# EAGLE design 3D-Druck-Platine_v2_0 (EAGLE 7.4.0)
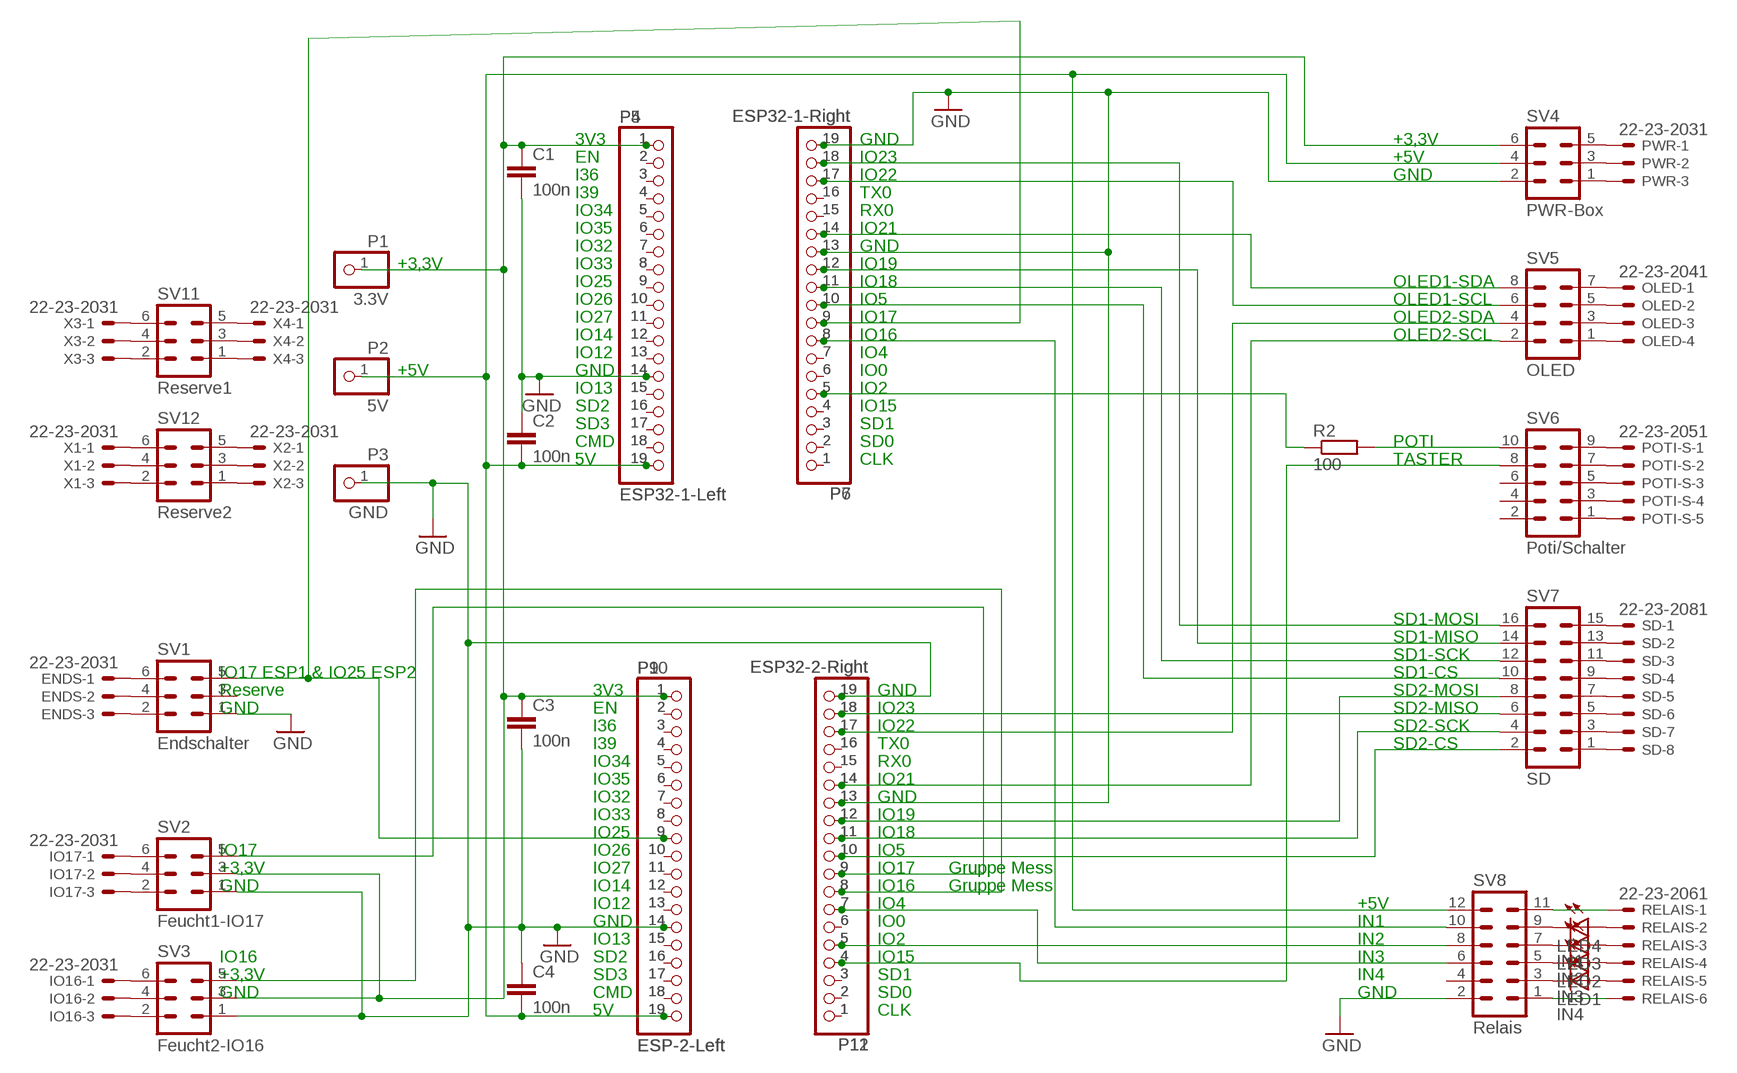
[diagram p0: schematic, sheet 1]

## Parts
C1  100n  C-EU025-024X044  [C025-024X044]
C2  100n  C-EU025-024X044  [C025-024X044]
C3  100n  C-EU025-024X044  [C025-024X044]
C4  100n  C-EU025-024X044  [C025-024X044]
ENDS  22-23-2031  [22-23-2031]
IO16  22-23-2031  [22-23-2031]
IO17  22-23-2031  [22-23-2031]
LED1  IN4  LED3MM  [LED3MM]
LED2  IN3  LED3MM  [LED3MM]
LED3  IN2  LED3MM  [LED3MM]
LED4  IN1  LED3MM  [LED3MM]
OLED  22-23-2041  [22-23-2041]
P1  3.3V  PINHD-1X1  [1X01]
P2  5V  PINHD-1X1  [1X01]
P3  GND  PINHD-1X1  [1X01]
P4  ESP32-1-Left  PINHD-1X19  [1X19]
P5  ESP32-1-Left  PINHD-1X19  [1X19]
P6  ESP32-1-Right  PINHD-1X19  [1X19]
P7  ESP32-1-Right  PINHD-1X19  [1X19]
P9  ESP-2-Left  PINHD-1X19  [1X19]
P10  ESP-2-Left  PINHD-1X19  [1X19]
P11  ESP32-2-Right  PINHD-1X19  [1X19]
P12  ESP32-2-Right  PINHD-1X19  [1X19]
POTI-S  22-23-2051  [22-23-2051]
PWR  22-23-2031  [22-23-2031]
R2  100  R-EU_0207/10  [0207/10]
RELAIS  22-23-2061  [22-23-2061]
SD  22-23-2081  [22-23-2081]
SV1  Endschalter  MA03-2  [MA03-2]
SV2  Feucht1-IO17  MA03-2  [MA03-2]
SV3  Feucht2-IO16  MA03-2  [MA03-2]
SV4  PWR-Box  MA03-2  [MA03-2]
SV5  OLED  MA04-2  [MA04-2]
SV6  Poti/Schalter  MA05-2  [MA05-2]
SV7  SD  MA08-2  [MA08-2]
SV8  Relais  MA06-2  [MA06-2]
SV11  Reserve1  MA03-2  [MA03-2]
SV12  Reserve2  MA03-2  [MA03-2]
X1  22-23-2031  [22-23-2031]
X2  22-23-2031  [22-23-2031]
X3  22-23-2031  [22-23-2031]
X4  22-23-2031  [22-23-2031]

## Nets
GND: C1.2 C2.1 C3.2 C4.1 P3.1 P4.14 P5.14 P6.13 P6.19 P7.13 P7.19 P9.14 P10.14 P11.13 P11.19 P12.13 P12.19 SV1.1 SV2.1 SV3.1 SV4.2 SV8.2
N$1: P4.2 P5.2
N$2: LED4.K(C) SV8.9
N$3: P4.3 P5.3
N$3V: C1.1 C3.1 P1.1 P4.1 P5.1 P9.1 P10.1 SV2.3 SV3.3 SV4.6
N$4: P11.8 P12.8 SV3.5
N$5: LED3.K(C) SV8.7
N$5V: C2.2 C4.2 P2.1 P4.19 P5.19 P9.19 P10.19 SV4.4 SV8.12
N$6: P4.4 P5.4
N$7: P4.5 P5.5
N$8: ENDS.1 SV1.6
N$9: P4.6 P5.6
N$10: IO17.1 SV2.6
N$11: ENDS.2 SV1.4
N$12: ENDS.3 SV1.2
N$13: IO17.2 SV2.4
N$14: IO17.3 SV2.2
N$15: IO16.1 SV3.6
N$16: IO16.2 SV3.4
N$17: IO16.3 SV3.2
N$18: PWR.1 SV4.5
N$19: PWR.2 SV4.3
N$20: LED2.K(C) SV8.5
N$21: P4.7 P5.7
N$22: P4.8 P5.8
N$23: P4.9 P5.9
N$24: P4.10 P5.10
N$25: P4.11 P5.11
N$26: P4.12 P5.12
N$27: P4.13 P5.13
N$28: P4.15 P5.15
N$29: P4.16 P5.16
N$30: P4.17 P5.17
N$31: P4.18 P5.18
N$32: P6.1 P7.1
N$33: P6.2 P7.2
N$34: P6.3 P7.3
N$35: P6.4 P7.4
N$36: PWR.3 SV4.1
N$37: P6.7 P7.7
N$38: P6.15 P7.15
N$39: P6.16 P7.16
N$40: P9.2 P10.2
N$41: P9.3 P10.3
N$42: P9.4 P10.4
N$43: P9.5 P10.5
N$44: P9.6 P10.6
N$45: P9.8 P10.8
N$46: P9.11 P10.11
N$47: P9.12 P10.12
N$48: P9.13 P10.13
N$49: P9.15 P10.15
N$50: P9.16 P10.16
N$51: P9.17 P10.17
N$52: P9.18 P10.18
N$53: P11.1 P12.1
N$54: P11.2 P12.2
N$55: P11.3 P12.3
N$56: OLED.1 SV5.7
N$57: P11.6 P12.6
N$58: P11.15 P12.15
N$59: R2.2 SV6.10
N$60: P6.6 P7.6
N$61: OLED.2 SV5.5
N$62: OLED.3 SV5.3
N$63: OLED.4 SV5.1
N$64: POTI-S.1 SV6.9
N$65: POTI-S.2 SV6.7
N$66: POTI-S.3 SV6.5
N$67: POTI-S.4 SV6.3
N$68: POTI-S.5 SV6.1
N$69: SD.1 SV7.15
N$70: SD.2 SV7.13
N$71: SD.3 SV7.11
N$72: SD.5 SV7.7
N$73: SD.6 SV7.5
N$74: SD.7 SV7.3
N$75: SD.8 SV7.1
N$76: SD.4 SV7.9
N$77: RELAIS.1 SV8.11
N$78: LED1.K(C) SV8.3
N$79: LED4.A RELAIS.2
N$80: LED3.A RELAIS.3
N$81: LED2.A RELAIS.4
N$82: RELAIS.6 SV8.1
N$83: LED1.A RELAIS.5
N$84: SV11.6 X3.1
N$85: SV11.4 X3.2
N$86: SV11.2 X3.3
N$87: SV11.5 X4.1
N$88: SV11.3 X4.2
N$89: SV11.1 X4.3
N$90: SV12.6 X1.1
N$91: SV12.4 X1.2
N$92: SV12.2 X1.3
N$93: SV12.5 X2.1
N$94: SV12.3 X2.2
N$95: SV12.1 X2.3
N$101: P11.16 P12.16
N$ESP1-18: P6.11 P7.11 SV7.12
N$ESP1-IO2: P6.5 P7.5 R2.1
N$ESP1-IO5: P6.10 P7.10 SV7.10
N$ESP1-IO16: P6.8 P7.8 SV8.10
N$ESP1-IO17_ESP2-IO25: P6.9 P7.9 P9.9 P10.9 SV1.5
N$ESP1-IO19: P6.12 P7.12 SV7.14
N$ESP1-IO21: P6.14 P7.14 SV5.8
N$ESP1-IO22: P6.17 P7.17 SV5.6
N$ESP1-IO23: P6.18 P7.18 SV7.16
N$ESP2-IO2: P11.5 P12.5 SV8.8
N$ESP2-IO4: P11.7 P12.7 SV8.6
N$ESP2-IO5: P11.10 P12.10 SV7.2
N$ESP2-IO15: P11.4 P12.4 SV6.8
N$ESP2-IO16: P11.9 P12.9 SV2.5
N$ESP2-IO18: P11.11 P12.11 SV7.4
N$ESP2-IO19: P11.12 P12.12 SV7.8
N$ESP2-IO21: P11.14 P12.14 SV5.2
N$ESP2-IO22: P11.17 P12.17 SV5.4
N$ESP2-IO23: P11.18 P12.18 SV7.6
N$ESP2-IO26: P9.10 P10.10
N$ESP2-IO32: P9.7 P10.7
Unconnected: SV1.3 SV6.2 SV6.4 SV6.6 SV8.4

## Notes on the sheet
- 3V3 | GND | +3,3V
- EN | IO23 | +5V
- I36 | IO22 | GND
- I39 | TX0
- IO34 | RX0
- IO35 | IO21
- IO32 | GND
- +3,3V | IO33 | IO19
- IO25 | IO18 | OLED1-SDA
- IO26 | IO5 | OLED1-SCL
- IO27 | IO17 | OLED2-SDA
- IO14 | IO16 | OLED2-SCL
- IO12 | IO4
- +5V | GND | IO0
- IO13 | IO2
- SD2 | IO15
- SD3 | SD1
- CMD | SD0 | POTI
- 5V | CLK | TASTER
- SD1-MOSI
- SD1-MISO
- SD1-SCK
- IO17 ESP1 & IO25 ESP2 | SD1-CS
- Reserve | 3V3 | GND | SD2-MOSI
- GND | EN | IO23 | SD2-MISO
- I36 | IO22 | SD2-SCK
- I39 | TX0 | SD2-CS
- IO34 | RX0
- IO35 | IO21
- IO32 | GND
- IO33 | IO19
- IO25 | IO18
- IO17 | IO26 | IO5
- +3,3V | IO27 | IO17 | Gruppe Mess
- GND | IO14 | IO16 | Gruppe Mess
- IO12 | IO4 | +5V
- GND | IO0 | IN1
- IO13 | IO2 | IN2
- IO16 | SD2 | IO15 | IN3
- +3,3V | SD3 | SD1 | IN4
- GND | CMD | SD0 | GND
- 5V | CLK

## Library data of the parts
C1-C4 = rcl:C-EU: CAPACITOR, European symbol
ENDS IO16 IO17 PWR X1-X4 = con-molex:22-23-2031: .100" (2.54mm) Center Header - 3 Pin; MF: MOLEX; MPN: 22-23-2031; OC_FARNELL: 1462950; OC_NEWARK: 30C0862
LED1-LED4 = led:LED: LED
OLED = con-molex:22-23-2041: .100" (2.54mm) Center Header - 4 Pin; MF: MOLEX; MPN: 22-23-2041; OC_FARNELL: 1462920; OC_NEWARK: 38C0355
P1-P3 = pinhead:PINHD-1X1: PIN HEADER
P4-P7 P9-P12 = pinhead:PINHD-1X19: PIN HEADER
POTI-S = con-molex:22-23-2051: .100" (2.54mm) Center Header - 5 Pin; MF: MOLEX; MPN: 22-23-2051; OC_FARNELL: 1462952; OC_NEWARK: 38C9178
R2 = rcl:R-EU_: RESISTOR, European symbol
RELAIS = con-molex:22-23-2061: .100" (2.54mm) Center Header - 6 Pin; MF: MOLEX; MPN: 22-23-2061; OC_FARNELL: 1462922; OC_NEWARK: 27C1933
SD = con-molex:22-23-2081: .100" (2.54mm) Center Header - 8 Pin; MF: MOLEX; MPN: 22-23-2081; OC_FARNELL: 1756826; OC_NEWARK: 01C7592
SV1-SV4 SV11 SV12 = con-lstb:MA03-2: PIN HEADER; OC_FARNELL: unknown; OC_NEWARK: unknown
SV5 = con-lstb:MA04-2: PIN HEADER; OC_FARNELL: unknown; OC_NEWARK: unknown
SV6 = con-lstb:MA05-2: PIN HEADER; OC_FARNELL: unknown; OC_NEWARK: unknown
SV7 = con-lstb:MA08-2: PIN HEADER; OC_FARNELL: unknown; OC_NEWARK: unknown
SV8 = con-lstb:MA06-2: PIN HEADER; OC_FARNELL: unknown; OC_NEWARK: unknown

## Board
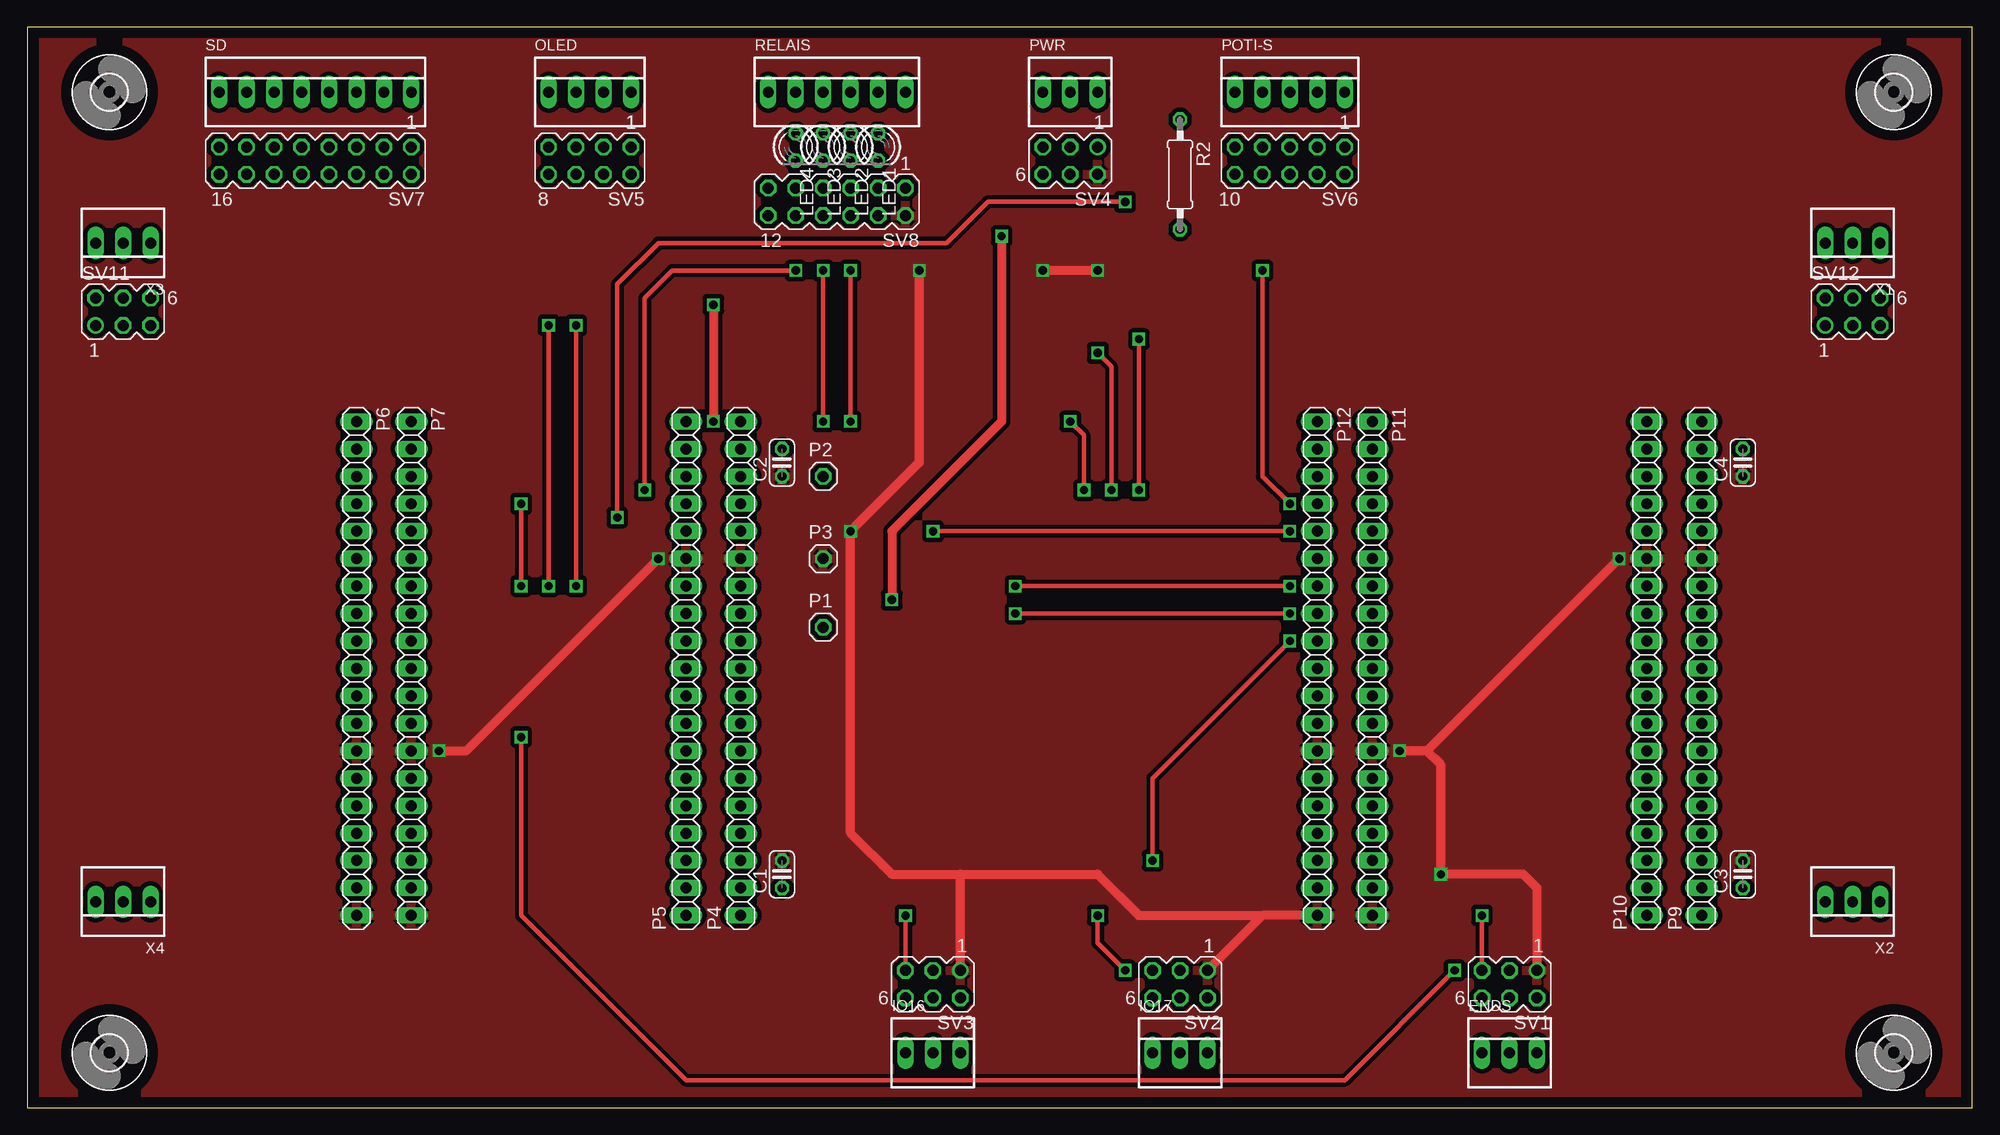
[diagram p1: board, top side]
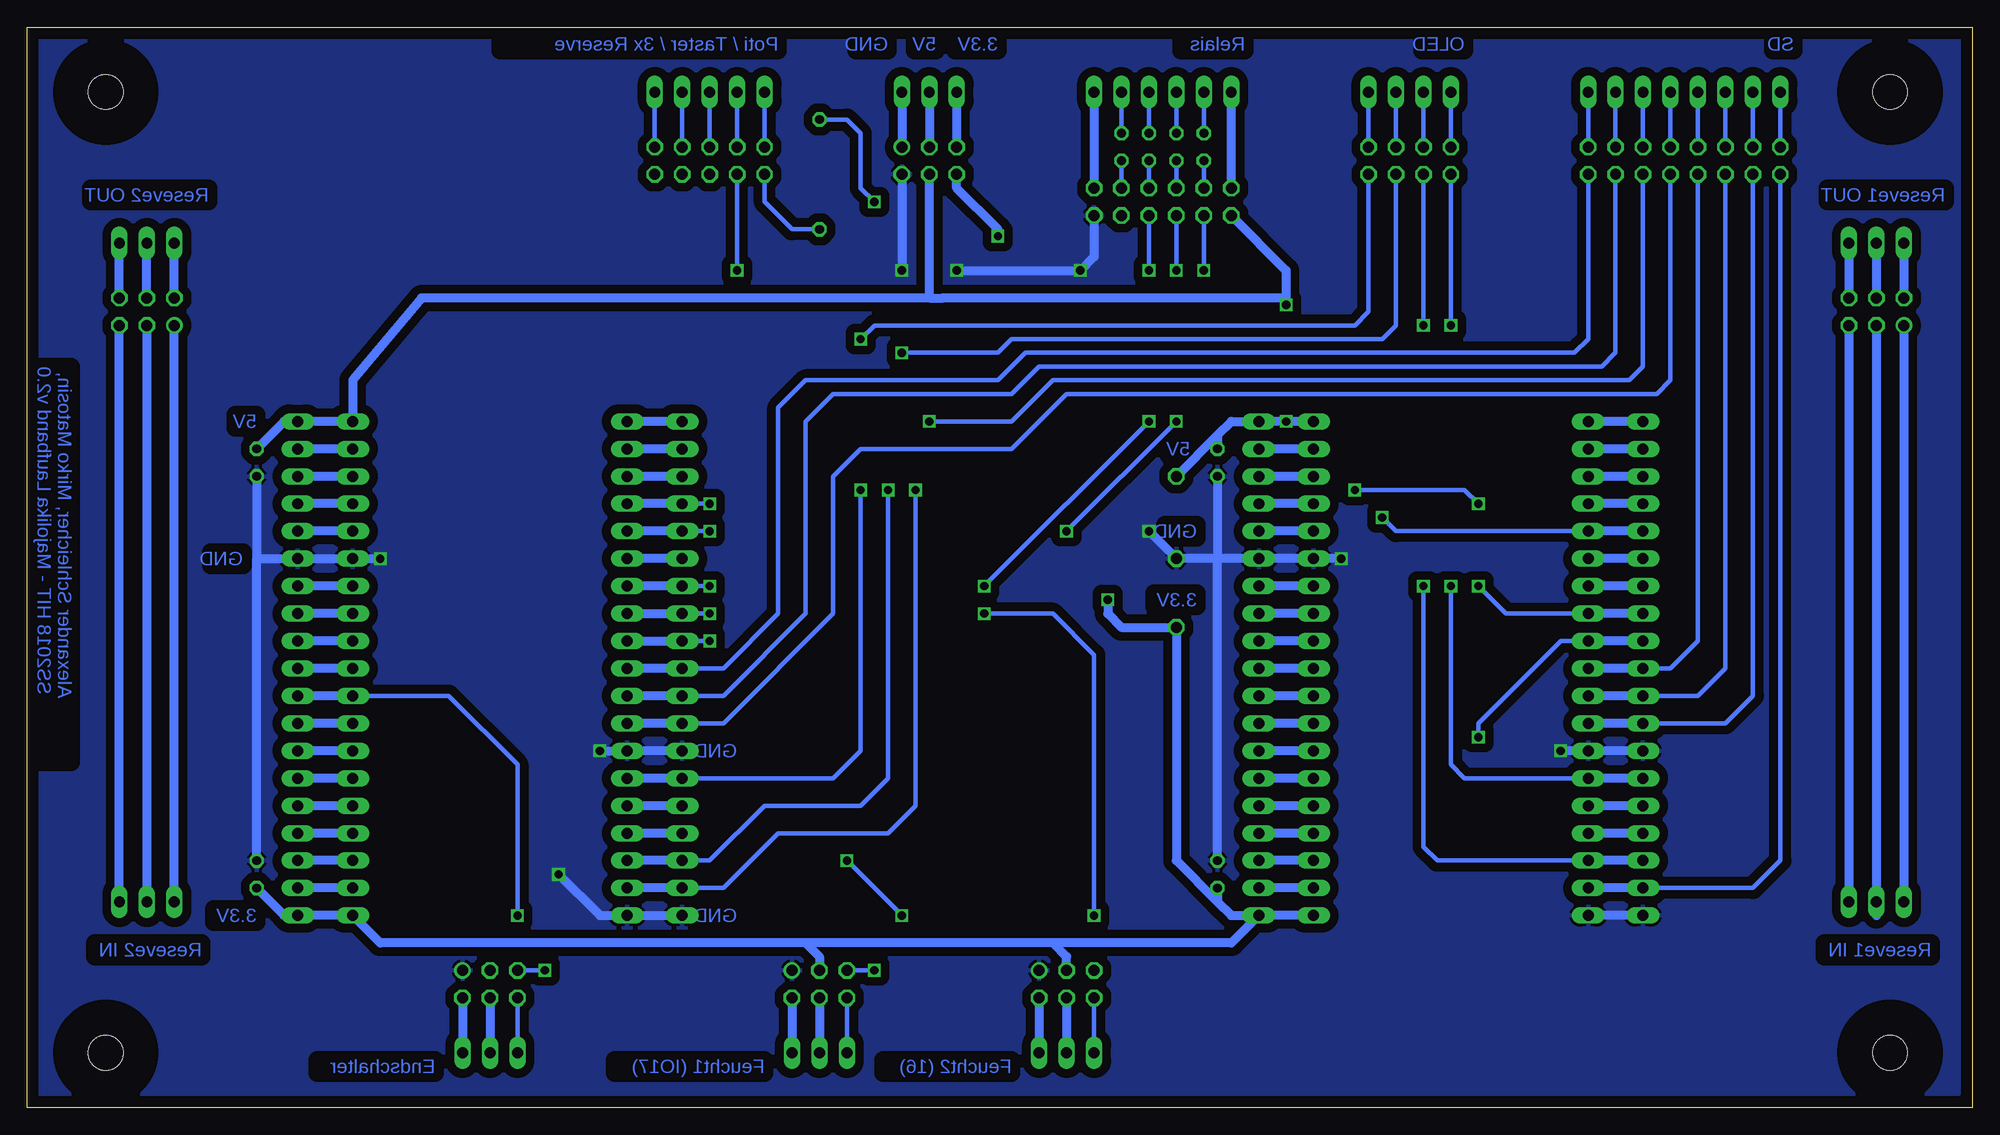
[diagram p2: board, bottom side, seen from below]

Size 180 x 100 mm. Coordinates in mm from the lower left corner, seen from the top.
Outline: 0,0 180,0 180,100 0,100 0,0
Copper layers (1*16): Top 0.035mm / dielectric 1.5mm / Bottom 0.035mm
Design rules "default": minimum track width 10mil, minimum drill 24mil, track to track 8mil, track to pad 8mil, pad to pad 8mil, via to via 8mil, smd to smd 8mil, copper to edge 40mil, drill to drill 8mil, minimum pad ring 10mil, minimum via ring 8mil, stop-mask expansion 4mil, vias tented up to drill 0mil, thermal gap 10mil

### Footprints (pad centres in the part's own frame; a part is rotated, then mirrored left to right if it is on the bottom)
C025-024X044 = drill 0.813 octagon: 1 -1.27,0; 2 1.27,0
22-23-2031 = drill 1 long: 1 -2.54,0; 2 0,0; 3 2.54,0
LED3MM = drill 0.813 octagon: A -1.27,0; K 1.27,0
22-23-2041 = drill 1 long: 1 -3.81,0; 2 -1.27,0; 3 1.27,0; 4 3.81,0
1X01 = drill 1.016 octagon: 1 0,0
1X19 = drill 1.016 long: 1 -22.86,0; 2 -20.32,0; 3 -17.78,0; 4 -15.24,0; 5 -12.7,0; 6 -10.16,0; 7 -7.62,0; 8 -5.08,0; 9 -2.54,0; 10 0,0; 11 2.54,0; 12 5.08,0; 13 7.62,0; 14 10.16,0; 15 12.7,0; 16 15.24,0; 17 17.78,0; 18 20.32,0; 19 22.86,0
22-23-2051 = drill 1 long: 1 -5.08,0; 2 -2.54,0; 3 0,0; 4 2.54,0; 5 5.08,0
0207/10 = drill 0.813 octagon: 1 -5.08,0; 2 5.08,0
22-23-2061 = drill 1 long: 1 -6.35,0; 2 -3.81,0; 3 -1.27,0; 4 1.27,0; 5 3.81,0; 6 6.35,0
22-23-2081 = drill 1 long: 1 -8.89,0; 2 -6.35,0; 3 -3.81,0; 4 -1.27,0; 5 1.27,0; 6 3.81,0; 7 6.35,0; 8 8.89,0
MA03-2 = drill 1.016: 1 -2.54,-1.27 | drill 1.016 octagon: 2 -2.54,1.27; 3 0,-1.27; 4 0,1.27; 5 2.54,-1.27; 6 2.54,1.27
MA04-2 = drill 1.016 octagon: 1 -3.81,-1.27; 2 -3.81,1.27; 3 -1.27,-1.27; 4 -1.27,1.27; 5 1.27,-1.27; 6 1.27,1.27; 7 3.81,-1.27; 8 3.81,1.27
MA05-2 = drill 1.016 octagon: 1 -5.08,-1.27; 2 -5.08,1.27; 3 -2.54,-1.27; 4 -2.54,1.27; 5 0,-1.27; 6 0,1.27; 7 2.54,-1.27; 8 2.54,1.27; 9 5.08,-1.27; 10 5.08,1.27
MA08-2 = drill 1.016 octagon: 1 -8.89,-1.27; 2 -8.89,1.27; 3 -6.35,-1.27; 4 -6.35,1.27; 5 -3.81,-1.27; 6 -3.81,1.27; 7 -1.27,-1.27; 8 -1.27,1.27; 9 1.27,-1.27; 10 1.27,1.27; 11 3.81,-1.27; 12 3.81,1.27; 13 6.35,-1.27; 14 6.35,1.27; 15 8.89,-1.27; 16 8.89,1.27
MA06-2 = drill 1.016 octagon: 1 -6.35,-1.27; 2 -6.35,1.27; 3 -3.81,-1.27; 4 -3.81,1.27; 5 -1.27,-1.27; 6 -1.27,1.27; 7 1.27,-1.27; 8 1.27,1.27; 9 3.81,-1.27; 10 3.81,1.27; 11 6.35,-1.27; 12 6.35,1.27
3,2 = hole 3.2: 0,0

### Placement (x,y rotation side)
C1  69.85,21.59 90 top
C2  69.85,59.69 90 top
C3  158.75,21.59 90 top
C4  158.75,59.69 90 top
ENDS  137.16,5.08 0 top
IO16  83.82,5.08 0 top
IO17  106.68,5.08 0 top
LED1  78.74,88.9 270 top
LED2  76.2,88.9 270 top
LED3  73.66,88.9 270 top
LED4  71.12,88.9 270 top
OLED  52.07,93.98 0 top
P1  73.66,44.45 0 top
P2  73.66,58.42 0 top
P3  73.66,50.8 0 top
P4  66.04,40.64 90 top
P5  60.96,40.64 90 top
P6  30.48,40.64 270 top
P7  35.56,40.64 270 top
P9  154.94,40.64 90 top
P10  149.86,40.64 90 top
P11  124.46,40.64 270 top
P12  119.38,40.64 270 top
POTI-S  116.84,93.98 0 top
PWR  96.52,93.98 0 top
R2  106.68,86.36 270 top
RELAIS  74.93,93.98 0 top
SD  26.67,93.98 0 top
SV1  137.16,11.43 180 top
SV2  106.68,11.43 180 top
SV3  83.82,11.43 180 top
SV4  96.52,87.63 180 top
SV5  52.07,87.63 180 top
SV6  116.84,87.63 180 top
SV7  26.67,87.63 180 top
SV8  74.93,83.82 180 top
SV11  8.89,73.66 0 top
SV12  168.91,73.66 0 top
U$1  [3,2]  7.62,93.98 0 top
U$2  [3,2]  7.62,5.08 0 top
U$3  [3,2]  172.72,93.98 0 top
U$4  [3,2]  172.72,5.08 0 top
X1  168.91,80.01 180 top
X2  168.91,19.05 180 top
X3  8.89,80.01 180 top
X4  8.89,19.05 180 top

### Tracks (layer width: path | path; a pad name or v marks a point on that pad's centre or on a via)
GND  (via drill 0.76)
  Top 0.813: v82.55,77.47 82.55,59.69 v76.2,53.34 76.2,25.4 80.01,21.59 86.36,21.59 | v99.06,77.47 v93.98,77.47 | v147.32,50.8 129.54,33.02 | 129.54,33.02 v127,33.02 | 129.54,33.02 130.81,31.75 v130.81,21.59 138.43,21.59 139.7,20.32 SV1.1 | SV3.1 86.36,21.59 | P12.19 114.3,17.78 | 114.3,17.78 SV2.1 | v38.1,33.02 40.64,33.02 v58.42,50.8 | 86.36,21.59 99.06,21.59 102.87,17.78 114.3,17.78
  Bottom 0.813: 69.85,50.8 P4.14 P5.14 v58.42,50.8 | 69.85,50.8 P3.1 v76.2,53.34 | P6.13 P7.13 v38.1,33.02 | P6.19 P7.19 | P12.13 P11.13 v127,33.02 | v93.98,77.47 v82.55,77.47 81.28,78.74 SV8.2 | v147.32,50.8 P10.14 P9.14 158.75,50.8 | v130.81,21.59 127,17.78 P11.19 P12.19 | C1.2 69.85,50.8 | C4.1 158.75,50.8 | C3.2 158.75,50.8 | C2.1 69.85,50.8 | SV4.2 v99.06,77.47
  pour Bottom (isolate 0.813): 1.27,99.06 179.07,99.06 179.07,87.63 179.07,1.27 1.27,1.27
  pour Top (isolate 0.406): 1.27,99.06 179.07,99.06 179.07,1.27 1.27,1.27
N$1
  Bottom 0.813: P5.2 P4.2
N$2
  Bottom 0.406: LED4.K SV8.9
N$3
  Bottom 0.813: P5.3 P4.3
N$3V  (via drill 0.76)
  Top 0.813: v90.17,80.64 90.17,63.5 80.01,53.34 v80.01,46.99
  Bottom 0.813: P5.1 P4.1 | v90.17,80.64 90.17,81.28 93.98,85.09 SV4.6 | 69.85,19.05 73.66,22.86 P1.1 78.74,44.45 80.01,45.72 v80.01,46.99 | 69.85,19.05 68.58,17.78 P4.1 | 85.09,15.24 68.58,15.24 P4.1 | 85.09,15.24 107.95,15.24 | 107.95,15.24 147.32,15.24 P10.1 P9.1 156.21,17.78 C3.1 | C1.1 69.85,19.05 | 107.95,15.24 106.68,13.97 SV2.3 | SV3.3 83.82,13.97 85.09,15.24
N$4  (via drill 0.76)
  Top 0.406: v91.44,45.72 v116.84,45.72 | v81.28,17.78 SV3.5
  Bottom 0.406: v91.44,45.72 85.09,45.72 81.28,41.91 v81.28,17.78 | v116.84,45.72 P12.8
  Bottom 0.813: P11.8 P12.8
N$5
  Bottom 0.406: LED3.K SV8.7
N$5V  (via drill 0.76)
  Top 0.813: v63.5,74.3 v63.5,63.5
  Bottom 0.813: 63.5,74.93 95.25,74.93 96.52,74.93 | 63.5,74.93 63.5,77.47 SV8.12 | 63.5,74.93 v63.5,74.3 | v63.5,63.5 P4.19 | P5.19 P4.19 | 96.52,74.93 143.51,74.93 149.86,67.31 P10.19 P9.19 156.21,63.5 C4.2 | P4.19 68.58,63.5 69.85,62.23 | 69.85,62.23 C2.2 | 96.52,74.93 SV4.4 | P2.1 69.85,62.23
N$6
  Bottom 0.813: P5.4 P4.4
N$7
  Bottom 0.813: P5.5 P4.5
N$8
  Bottom 0.406: SV1.6 ENDS.1
N$9
  Bottom 0.813: P5.6 P4.6
N$10
  Bottom 0.406: SV2.6 IO17.1
N$11
  Bottom 0.813: SV1.4 ENDS.2
N$12
  Bottom 0.813: SV1.2 ENDS.3
N$13
  Bottom 0.813: SV2.4 IO17.2
N$14
  Bottom 0.813: SV2.2 IO17.3
N$15
  Bottom 0.406: SV3.6 IO16.1
N$16
  Bottom 0.813: SV3.4 IO16.2
N$17
  Bottom 0.813: SV3.2 IO16.3
N$18
  Bottom 0.813: PWR.1 SV4.5
N$19
  Bottom 0.813: PWR.2 SV4.3
N$20
  Bottom 0.406: LED2.K SV8.5
N$21
  Bottom 0.813: P5.7 P4.7
N$22
  Bottom 0.813: P5.8 P4.8
N$23
  Bottom 0.813: P5.9 P4.9
N$24
  Bottom 0.813: P5.10 P4.10
N$25
  Bottom 0.813: P5.11 P4.11
N$26
  Bottom 0.813: P5.12 P4.12
N$27
  Bottom 0.813: P5.13 P4.13
N$28
  Bottom 0.813: P5.15 P4.15
N$29
  Bottom 0.813: P5.16 P4.16
N$30
  Bottom 0.813: P5.17 P4.17
N$31
  Bottom 0.813: P5.18 P4.18
N$32
  Bottom 0.813: P6.1 P7.1
N$33
  Bottom 0.813: P6.2 P7.2
N$34
  Bottom 0.813: P6.3 P7.3
N$35
  Bottom 0.813: P6.4 P7.4
N$36
  Bottom 0.813: PWR.3 SV4.1
N$37
  Bottom 0.813: P6.7 P7.7
N$38
  Bottom 0.813: P6.15 P7.15
N$39
  Bottom 0.813: P6.16 P7.16
N$40
  Bottom 0.813: P10.2 P9.2
N$41
  Bottom 0.813: P10.3 P9.3
N$42
  Bottom 0.813: P10.4 P9.4
N$43
  Bottom 0.813: P10.5 P9.5
N$44
  Bottom 0.813: P10.6 P9.6
N$45
  Bottom 0.813: P10.8 P9.8
N$46
  Bottom 0.813: P10.11 P9.11
N$47
  Bottom 0.813: P10.12 P9.12
N$48
  Bottom 0.813: P10.13 P9.13
N$49
  Bottom 0.813: P10.15 P9.15
N$50
  Bottom 0.813: P10.16 P9.16
N$51
  Bottom 0.813: P10.17 P9.17
N$52
  Bottom 0.813: P10.18 P9.18
N$53
  Bottom 0.813: P12.1 P11.1
N$54
  Bottom 0.813: P12.2 P11.2
N$55
  Bottom 0.813: P12.3 P11.3
N$56
  Bottom 0.406: OLED.1 SV5.7
N$57
  Bottom 0.813: P12.6 P11.6
N$58
  Bottom 0.813: P12.15 P11.15
N$59
  Bottom 0.406: R2.2 109.22,81.28 111.76,83.82 SV6.10
N$60
  Bottom 0.813: P6.6 P7.6
N$61
  Bottom 0.406: OLED.2 SV5.5
N$62
  Bottom 0.406: OLED.3 SV5.3
N$63
  Bottom 0.406: OLED.4 SV5.1
N$64
  Bottom 0.406: POTI-S.1 SV6.9
N$65
  Bottom 0.406: POTI-S.2 SV6.7
N$66
  Bottom 0.406: POTI-S.3 SV6.5
N$67
  Bottom 0.406: POTI-S.4 SV6.3
N$68
  Bottom 0.406: POTI-S.5 SV6.1
N$69
  Bottom 0.406: SD.1 SV7.15
N$70
  Bottom 0.406: SD.2 SV7.13
N$71
  Bottom 0.406: SD.3 SV7.11
N$72
  Bottom 0.406: SD.5 SV7.7
N$73
  Bottom 0.406: SD.6 SV7.5
N$74
  Bottom 0.406: SD.7 SV7.3
N$75
  Bottom 0.406: SD.8 SV7.1
N$76
  Bottom 0.406: SD.4 SV7.9
N$77
  Bottom 0.813: SV8.11 RELAIS.1
N$78
  Bottom 0.406: LED1.K SV8.3
N$79
  Bottom 0.406: RELAIS.2 LED4.A
N$80
  Bottom 0.406: RELAIS.3 LED3.A
N$81
  Bottom 0.406: RELAIS.4 LED2.A
N$82
  Bottom 0.813: RELAIS.6 SV8.1
N$83
  Bottom 0.406: RELAIS.5 LED1.A
N$84
  Bottom 0.813: X3.1 SV11.6
N$85
  Bottom 0.813: X3.2 SV11.4
N$86
  Bottom 0.813: X3.3 SV11.2
N$87
  Bottom 0.813: SV11.5 X4.1
N$88
  Bottom 0.813: SV11.3 X4.2 8.89,17.78
N$89
  Bottom 0.813: SV11.1 X4.3
N$90
  Bottom 0.813: SV12.6 X1.1
N$91
  Bottom 0.813: SV12.4 X1.2
N$92
  Bottom 0.813: SV12.2 X1.3
N$93
  Bottom 0.813: X2.1 SV12.5
N$94
  Bottom 0.813: SV12.3 X2.2
N$95
  Bottom 0.813: X2.3 SV12.1
N$101
  Bottom 0.813: P12.16 P11.16
N$ESP1-18
  Bottom 0.406: P6.11 25.4,38.1 22.86,40.64 SV7.12
  Bottom 0.813: P6.11 P7.11
N$ESP1-IO2  (via drill 0.76)
  Top 0.406: v101.6,83.82 88.9,83.82 85.09,80.01 58.42,80.01 54.61,76.2 v54.61,54.61
  Bottom 0.406: R2.1 104.14,91.44 102.87,90.17 102.87,85.09 v101.6,83.82 | P7.5 53.34,53.34 v54.61,54.61
  Bottom 0.813: P6.5 P7.5
N$ESP1-IO5
  Bottom 0.406: P6.10 27.94,40.64 25.4,43.18 SV7.10
  Bottom 0.813: P6.10 P7.10
N$ESP1-IO16  (via drill 0.76)
  Top 0.406: v71.12,77.47 59.69,77.47 57.15,74.93 v57.15,57.15 | v45.72,55.88 v45.72,48.26
  Bottom 0.406: P7.8 43.18,45.72 v45.72,48.26 | v71.12,77.47 SV8.10 | v57.15,57.15 46.99,57.15 v45.72,55.88
  Bottom 0.813: P6.8 P7.8
N$ESP1-IO17_ESP2-IO25  (via drill 0.76)
  Top 0.406: v45.72,34.29 45.72,17.78 60.96,2.54 121.92,2.54 v132.08,12.7 | v134.62,17.78 SV1.5
  Bottom 0.406: P10.9 140.97,38.1 134.62,31.75 v134.62,17.78 | P7.9 38.1,43.18 45.72,35.56 v45.72,34.29 | v132.08,12.7 SV1.5
  Bottom 0.813: P6.9 P7.9 | P10.9 P9.9
N$ESP1-IO19
  Bottom 0.406: P6.12 22.86,35.56 20.32,38.1 SV7.14
  Bottom 0.813: P6.12 P7.12
N$ESP1-IO21  (via drill 0.76)
  Top 0.406: v48.26,72.39 v48.26,48.26
  Bottom 0.406: v48.26,48.26 48.26,31.75 46.99,30.48 P7.14 | v48.26,72.39 SV5.8
  Bottom 0.813: P6.14 P7.14
N$ESP1-IO22  (via drill 0.76)
  Top 0.406: v50.8,72.39 v50.8,48.26
  Bottom 0.406: v50.8,48.26 50.8,24.13 49.53,22.86 P7.17 | v50.8,72.39 SV5.6
  Bottom 0.813: P6.17 P7.17
N$ESP1-IO23
  Bottom 0.406: P6.18 20.32,20.32 17.78,22.86 SV7.16
  Bottom 0.813: P6.18 P7.18
N$ESP2-IO2  (via drill 0.76)
  Top 0.406: v73.66,77.47 v73.66,63.5 | v83.82,53.34 v116.84,53.34
  Bottom 0.406: v73.66,63.5 v83.82,53.34 | v116.84,53.34 P12.5 | v73.66,77.47 SV8.8
  Bottom 0.813: P12.5 P11.5
N$ESP2-IO4  (via drill 0.76)
  Top 0.406: v76.2,77.47 v76.2,63.5 | v91.44,48.26 v116.84,48.26
  Bottom 0.406: v76.2,63.5 v91.44,48.26 | v116.84,48.26 P12.7 | v76.2,77.47 SV8.6
  Bottom 0.813: P12.7 P11.7
N$ESP2-IO5
  Bottom 0.406: P12.10 115.57,40.64 110.49,45.72 110.49,64.77 107.95,67.31 90.17,67.31 87.63,69.85 36.83,69.85 35.56,71.12 SV7.2
  Bottom 0.813: P12.10 P11.10
N$ESP2-IO15  (via drill 0.76)
  Top 0.406: v114.3,77.47 114.3,58.42 v116.84,55.88
  Bottom 0.406: v116.84,55.88 P12.4 | v114.3,77.47 SV6.8
  Bottom 0.813: P12.4 P11.4
N$ESP2-IO16  (via drill 0.76)
  Top 0.406: v116.84,43.18 104.14,30.48 v104.14,22.86 | v99.06,17.78 99.06,15.24 v101.6,12.7
  Bottom 0.406: P12.9 v116.84,43.18 | v104.14,22.86 v99.06,17.78 | v101.6,12.7 SV2.5
  Bottom 0.813: P11.9 P12.9
N$ESP2-IO18
  Bottom 0.406: P12.11 115.57,38.1 107.95,45.72 107.95,63.5 105.41,66.04 88.9,66.04 86.36,68.58 34.29,68.58 33.02,69.85 SV7.4
  Bottom 0.813: P12.11 P11.11
N$ESP2-IO19
  Bottom 0.406: P12.12 115.57,35.56 105.41,45.72 105.41,58.42 102.87,60.96 88.9,60.96 83.82,66.04 29.21,66.04 27.94,67.31 SV7.8
  Bottom 0.813: P12.12 P11.12
N$ESP2-IO21  (via drill 0.76)
  Top 0.406: v102.87,71.12 v102.87,57.15
  Bottom 0.406: v102.87,71.12 101.6,72.39 57.15,72.39 55.88,73.66 SV5.2 | v102.87,57.15 102.87,33.02 105.41,30.48 P12.14
  Bottom 0.813: P12.14 P11.14
N$ESP2-IO22  (via drill 0.76)
  Top 0.406: v99.06,69.85 100.33,68.58 v100.33,57.15
  Bottom 0.406: v100.33,57.15 100.33,30.48 102.87,27.94 111.76,27.94 116.84,22.86 P12.17 | SV5.4 53.34,72.39 54.61,71.12 88.9,71.12 90.17,69.85 v99.06,69.85
  Bottom 0.813: P12.17 P11.17
N$ESP2-IO23  (via drill 0.76)
  Top 0.406: v96.52,63.5 97.79,62.23 v97.79,57.15
  Bottom 0.406: v97.79,57.15 97.79,27.94 100.33,25.4 110.49,25.4 115.57,20.32 P12.18 | SV7.6 30.48,68.58 31.75,67.31 85.09,67.31 88.9,63.5 v96.52,63.5
  Bottom 0.813: P12.18 P11.18
N$ESP2-IO26
  Bottom 0.813: P10.10 P9.10
N$ESP2-IO32
  Bottom 0.813: P10.7 P9.7

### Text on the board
Bottom: SD | OLED | Relais | 3.3V | 5V | GND | Poti / Taster / 3x Reserve | Reseve1 OUT | Reseve2 OUT | Alexander Schleicher, Mirko Matosin, / SS2018 HIT - Majolika Laufband v2.0 | 5V | 5V | GND | GND | 3.3V | GND | GND | 3.3V | Reseve1 IN | Reseve2 IN | Feucht2 (16) | Feucht1 (IO17) | Endschalter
